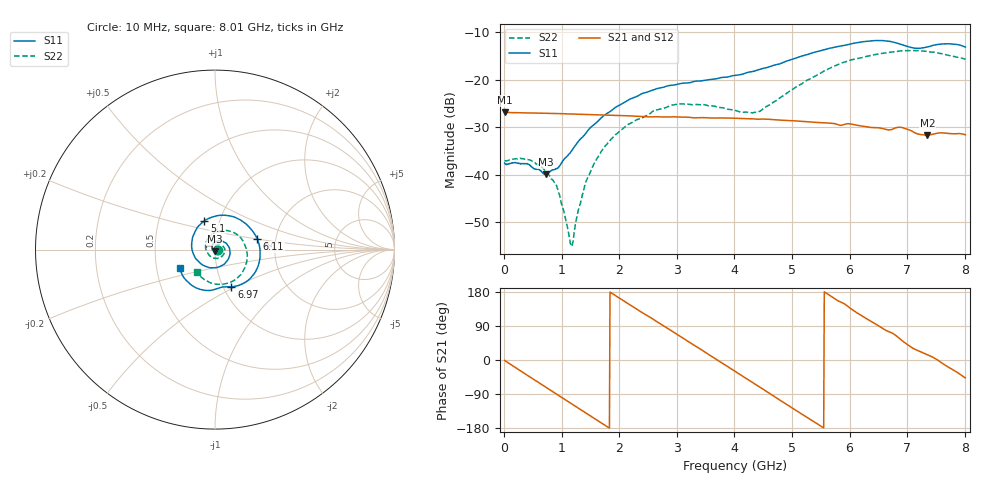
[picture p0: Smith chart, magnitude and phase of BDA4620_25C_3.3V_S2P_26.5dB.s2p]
!Agilent Technologies,E5071B,MY42404982,A.09.10
!Date: Wed May 06 08:54:34 2026
!Data & Calibration Information:
!Freq	S11:SOLT2(ON)	S21:SOLT2(ON)	S12:SOLT2(ON)	S22:SOLT2(ON)
# Hz S RI R 50
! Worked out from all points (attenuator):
!   801 points, 10 MHz to 8.01 GHz, reference 50 ohm
!   highest |S21| = -26.87 dB at 10 MHz (marker M1); lowest = -31.7 dB at 7.35 GHz (marker M2)
!   lowest |S11| = -39.9 dB at 720 MHz (marker M3), VSWR 1.02, Z = 49.8 - j0.993 ohm
!   |S11| at or under -10 dB: start of sweep to end of sweep
!   |S22| runs from -55.0 to -13.9 dB; largest |S21 - S12| = 0.00021
!   S11 on the Smith chart (normalised r, x): 10 MHz: 1.03, -0.00; 5.1 GHz: 0.85, +0.28; 6.11 GHz: 1.60, +0.20; 6.97 GHz: 1.09, -0.48; 8.01 GHz: 0.66, -0.14
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1e7  0.0133 -0.000814  0.0453 -0.000951  0.0453 -0.000944  0.0139 -0.000445
4.3e8  0.00868 -0.00953  0.0327 -0.0304  0.0327 -0.0305  0.0135 -0.00505
7.2e8  -0.00195 -0.00997  0.0141 -0.042  0.0141 -0.042  0.00852 -0.00723
9.3e8  -0.0104 -0.0054  -0.00156 -0.0439  -0.00166 -0.044  0.00356 -0.00618
1.16e9  -0.0164 0.00571  -0.0181 -0.0395  -0.0182 -0.0396  -0.00144 -0.00118
1.2e9  -0.017 0.00807  -0.0208 -0.0382  -0.0208 -0.0382  -0.002 1.56e-05
1.35e9  -0.0172 0.0176  -0.0296 -0.0314  -0.0296 -0.0315  -0.00354 0.00457
1.53e9  -0.0127 0.0299  -0.0373 -0.0209  -0.0374 -0.021  -0.00337 0.0112
1.77e9  0.00149 0.0432  -0.0421 -0.00445  -0.0422 -0.00444  0.000704 0.0205
2.15e9  0.0374 0.0477  -0.0358 0.0214  -0.0358 0.0215  0.0169 0.0292
2.68e9  0.0808 0.006  -0.00617 0.0401  -0.00615 0.0402  0.0442 0.0195
3.08e9  0.0755 -0.0509  0.0201 0.035  0.0202 0.035  0.0551 -0.0072
4.01e9  -0.073 -0.0832  0.034 -0.0195  0.0341 -0.0195  -0.0102 -0.0464
4.42e9  -0.1269 -0.00467  0.0135 -0.036  0.0135 -0.036  -0.0443 -0.0128
5.1e9  -0.0586 0.1603  -0.0263 -0.0255  -0.0265 -0.0255  -0.0184 0.0841
5.35e9  0.0158 0.1897  -0.0337 -0.0121  -0.0336 -0.0122  0.0229 0.1018
6.11e9  0.2356 0.0589  -0.0197 0.0269  -0.0197 0.0269  0.1601 0.04
6.68e9  0.1892 -0.1674  0.0078 0.0285  0.0078 0.0286  0.1701 -0.09
6.97e9  0.0912 -0.2067  0.0218 0.0213  0.0219 0.0214  0.1307 -0.1528
7.35e9  0.00516 -0.2201  0.0253 0.00628  0.0254 0.00631  0.0403 -0.1932
7.66e9  -0.1057 -0.2131  0.0267 -0.00651  0.0267 -0.00655  -0.0351 -0.1801
8.01e9  -0.1951 -0.1005  0.0179 -0.0193  0.018 -0.0193  -0.1017 -0.1273
